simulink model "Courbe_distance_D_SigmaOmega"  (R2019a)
settings: Solver=VariableStepAuto  StartTime=0.0  StopTime=6.283185307  MaxStep=0.001  RelTol=1e-6  SampleTimeConstraint=STIndependent

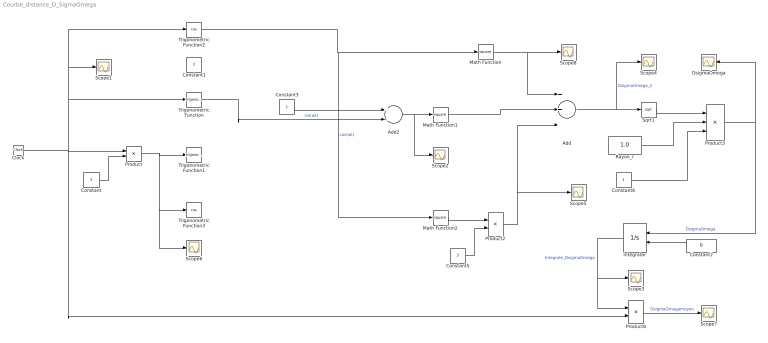
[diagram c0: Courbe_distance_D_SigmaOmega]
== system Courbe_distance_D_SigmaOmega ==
  Add : Sum  Inputs=+++
  Add2 : Sum  Inputs=+-
  Clock : Clock
  Constant : Constant  Value=3
  Constant1 : Constant  Value=2
  Constant2 : Constant  Value=0
  Constant3 : Constant
  Constant5 : Constant  Value=3
  Constant6 : Constant
  DsigmaOmega : Scope
  Integrator : Integrator  InitialConditionSource=external
  Math Function : Math  Operator=square
  Math Function1 : Math  Operator=square
  Math Function2 : Math  Operator=square
  Product : Product
  Product2 : Product
  Product3 : Product  Inputs=**/
  Product8 : Product  Inputs=*/
  Rayon_r : Constant  Value=1.0
  Scope{1..8} (8 alike) : Scope
  Sqrt1 : Sqrt
  Trigonometric Function : Trigonometry
  Trigonometric Function1 : Trigonometry
  Trigonometric Function2 : Trigonometry  Operator=cos
  Trigonometric Function3 : Trigonometry  Operator=cos
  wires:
  Product/1 -> Scope6/1, Trigonometric Function3/1, Trigonometric Function1/1
  Constant/1 -> Product/2
  Clock/1 -> Product8/2, Trigonometric Function/1, Trigonometric Function2/1, Scope1/1, Product/1
  Add2/1 -> Scope2/1, Math Function1/1
  Math Function/1 -> Scope8/1, Add/1
  Add/1 -> Sqrt1/1, Scope4/1  "DsigmaOmega_2"
  Integrator/1 -> Product8/1, Scope3/1  "Integrale_DsigmaOmega"
  Constant2/1 -> Integrator/2
  Product8/1 -> Scope7/1  "DsigmaOmegamoyen"
  Constant5/1 -> Product2/2
  Product2/1 -> Add/3, Scope5/1
  Sqrt1/1 -> Product3/1
  Rayon_r/1 -> Product3/2
  Constant6/1 -> Product3/3
  Product3/1 -> Integrator/1, DsigmaOmega/1  "DsigmaOmega"
  Constant3/1 -> Add2/1
  Math Function1/1 -> Add/2
  Math Function2/1 -> Product2/1
  Trigonometric Function2/1 -> Math Function2/1, Math Function/1  "cos(wt)"
  Trigonometric Function/1 -> Add2/2  "sin(wt)"
